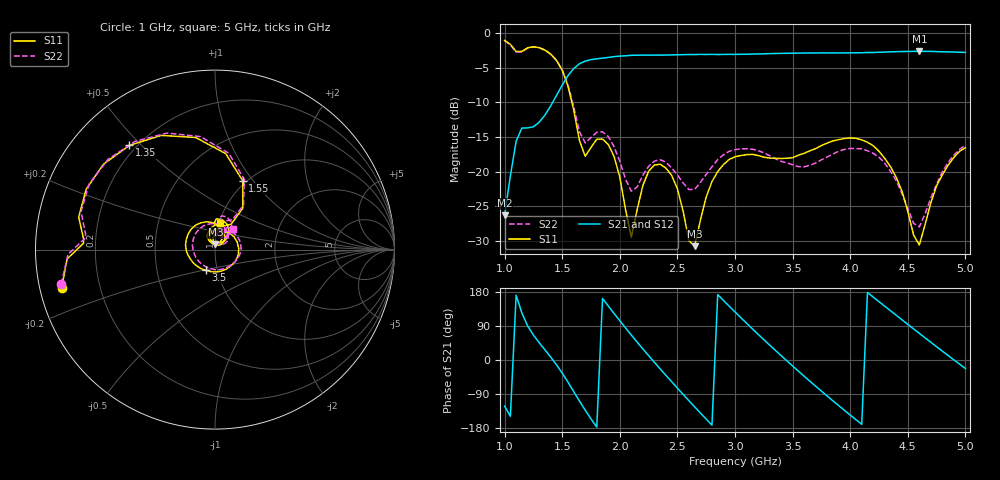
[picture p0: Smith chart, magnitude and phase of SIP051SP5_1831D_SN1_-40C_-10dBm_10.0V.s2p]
# GHz  S  dB  R  50
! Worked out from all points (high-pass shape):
!   81 points, 1 GHz to 5 GHz, reference 50 ohm
!   highest |S21| = -2.66 dB at 4.6 GHz (marker M1); lowest = -26.3 dB at 1 GHz (marker M2)
!   |S21| within 3 dB of the highest: 1.575 GHz to end of sweep
!   lowest |S11| = -30.7 dB at 2.65 GHz (marker M3), VSWR 1.06, Z = 50.2 + j2.91 ohm
!   |S11| at or under -10 dB: 1.584 GHz to end of sweep
!   |S22| runs from -27.9 to -1.1 dB; largest |S21 - S12| = 0.0019
!   S11 on the Smith chart (normalised r, x): 1 GHz: 0.06, -0.12; 1.35 GHz: 0.17, +0.46; 1.55 GHz: 0.96, +0.89; 3.5 GHz: 0.88, -0.21; 5 GHz: 1.01, +0.30
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1  -1.10 -165.9  -26.29 -121.6  -26.22 -122.0  -1.13 -167.3
1.1  -2.69 177.3  -15.62 170.8  -15.64 170.9  -2.79 174.9
1.35  -2.48 129.4  -11.85 26.8  -11.85 26.7  -2.50 126.5
1.55  -7.68 68.0  -6.17 -58.4  -6.16 -58.3  -7.48 67.3
1.7  -17.80 78.9  -4.07 -132.6  -4.07 -132.6  -15.87 75.2
1.85  -15.30 76.8  -3.65 162.3  -3.64 162.4  -14.25 70.5
2.05  -25.48 47.2  -3.31 84.6  -3.29 84.6  -21.08 48.6
2.1  -29.43 84.6  -3.24 65.8  -3.24 65.9  -22.81 62.9
2.2  -22.00 112.7  -3.21 29.3  -3.21 29.4  -20.50 81.9
2.35  -18.92 79.1  -3.22 -23.3  -3.20 -23.2  -18.27 64.7
2.5  -22.46 43.8  -3.17 -74.2  -3.16 -74.2  -20.47 46.3
2.65  -30.73 84.7  -3.13 -123.7  -3.12 -123.8  -22.56 60.1
2.8  -21.43 91.0  -3.11 -171.8  -3.10 -171.9  -19.29 62.8
3  -17.85 33.6  -3.11 126.8  -3.10 126.7  -16.84 31.6
3.2  -17.66 -28.9  -3.04 68.0  -3.04 68.0  -16.96 -9.2
3.5  -17.99 -113.7  -2.94 -15.8  -2.94 -15.8  -19.00 -89.9
3.7  -16.68 -158.6  -2.91 -69.0  -2.90 -69.1  -18.75 -159.2
4.05  -15.19 128.8  -2.88 -157.5  -2.88 -157.6  -16.68 103.3
4.35  -19.28 69.0  -2.74 129.9  -2.76 129.9  -19.94 42.6
4.6  -30.56 95.3  -2.67 70.3  -2.67 70.3  -27.95 66.4
4.8  -20.45 115.7  -2.73 23.4  -2.73 23.4  -20.03 80.8
5  -16.55 78.9  -2.82 -22.4  -2.83 -22.4  -16.18 48.6
